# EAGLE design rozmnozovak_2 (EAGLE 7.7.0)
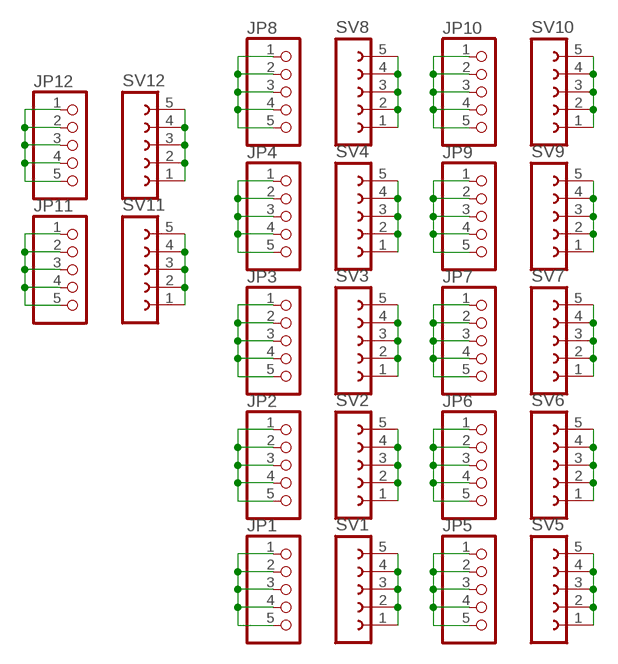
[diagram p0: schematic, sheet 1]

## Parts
JP1  PINHD-1X5  [1X05]
JP2  PINHD-1X5  [1X05]
JP3  PINHD-1X5  [1X05]
JP4  PINHD-1X5  [1X05]
JP5  PINHD-1X5  [1X05]
JP6  PINHD-1X5  [1X05]
JP7  PINHD-1X5  [1X05]
JP8  PINHD-1X5  [1X05]
JP9  PINHD-1X5  [1X05]
JP10  PINHD-1X5  [1X05]
JP11  PINHD-1X5  [1X05]
JP12  PINHD-1X5  [1X05]
SV1  FE05-1  [FE05-1]
SV2  FE05-1  [FE05-1]
SV3  FE05-1  [FE05-1]
SV4  FE05-1  [FE05-1]
SV5  FE05-1  [FE05-1]
SV6  FE05-1  [FE05-1]
SV7  FE05-1  [FE05-1]
SV8  FE05-1  [FE05-1]
SV9  FE05-1  [FE05-1]
SV10  FE05-1  [FE05-1]
SV11  FE05-1  [FE05-1]
SV12  FE05-1  [FE05-1]

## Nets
N$1: SV4.1 SV4.2 SV4.3 SV4.4 SV4.5
N$2: SV3.1 SV3.2 SV3.3 SV3.4 SV3.5
N$3: SV2.1 SV2.2 SV2.3 SV2.4 SV2.5
N$4: SV1.1 SV1.2 SV1.3 SV1.4 SV1.5
N$5: JP4.1 JP4.2 JP4.3 JP4.4 JP4.5
N$6: JP3.1 JP3.2 JP3.3 JP3.4 JP3.5
N$7: JP2.1 JP2.2 JP2.3 JP2.4 JP2.5
N$8: JP1.1 JP1.2 JP1.3 JP1.4 JP1.5
N$9: SV9.1 SV9.2 SV9.3 SV9.4 SV9.5
N$10: SV7.1 SV7.2 SV7.3 SV7.4 SV7.5
N$11: SV6.1 SV6.2 SV6.3 SV6.4 SV6.5
N$12: SV5.1 SV5.2 SV5.3 SV5.4 SV5.5
N$13: JP9.1 JP9.2 JP9.3 JP9.4 JP9.5
N$14: SV8.1 SV8.2 SV8.3 SV8.4 SV8.5
N$15: JP8.1 JP8.2 JP8.3 JP8.4 JP8.5
N$16: JP7.1 JP7.2 JP7.3 JP7.4 JP7.5
N$17: JP6.1 JP6.2 JP6.3 JP6.4 JP6.5
N$18: JP5.1 JP5.2 JP5.3 JP5.4 JP5.5
N$19: SV10.1 SV10.2 SV10.3 SV10.4 SV10.5
N$20: JP10.1 JP10.2 JP10.3 JP10.4 JP10.5
N$21: SV11.1 SV11.2 SV11.3 SV11.4 SV11.5
N$22: JP11.1 JP11.2 JP11.3 JP11.4 JP11.5
N$23: SV12.1 SV12.2 SV12.3 SV12.4 SV12.5
N$24: JP12.1 JP12.2 JP12.3 JP12.4 JP12.5

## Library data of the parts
JP1-JP12 = pinhead:PINHD-1X5: PIN HEADER
SV1-SV12 = con-lsta:FE05-1: FEMALE HEADER; OC_FARNELL: unknown; OC_NEWARK: unknown

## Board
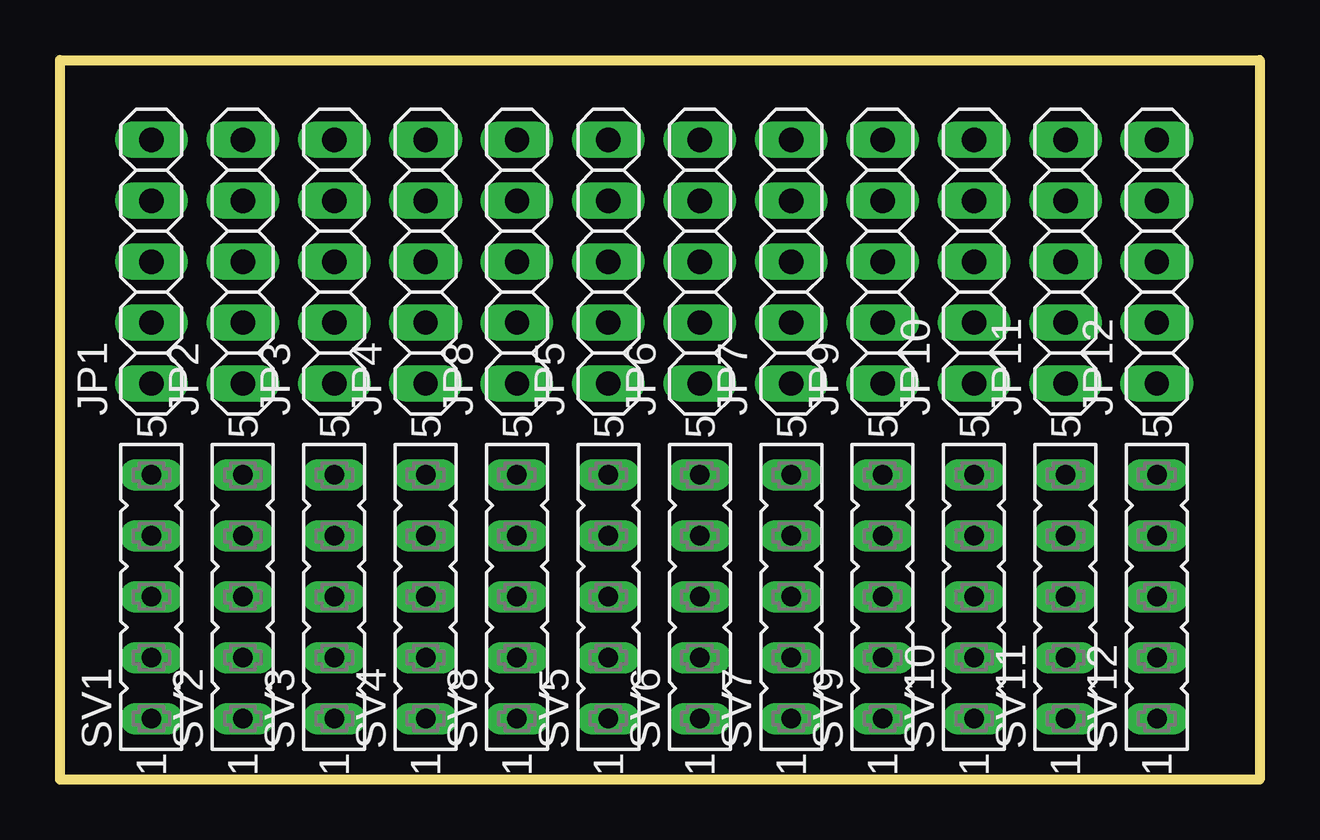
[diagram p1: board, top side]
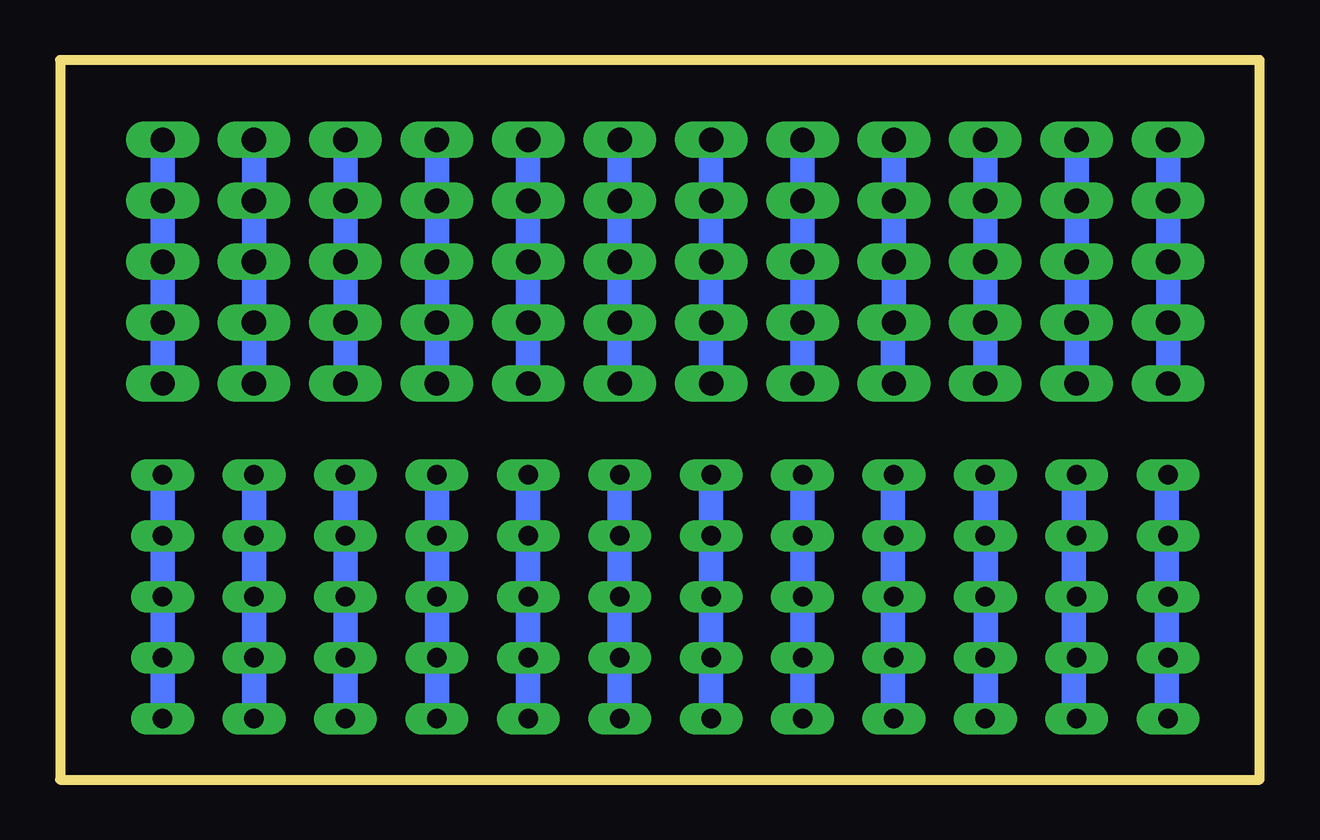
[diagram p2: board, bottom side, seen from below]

Size 50 x 30 mm. Coordinates in mm from the lower left corner, seen from the top.
Outline: 0,0 0,30 50,30 50,0 0,0
Copper layers (1*16): Top 0.035mm / dielectric 1.5mm / Bottom 0.035mm
Design rules "default": minimum track width 10mil, minimum drill 24mil, track to track 8mil, track to pad 8mil, pad to pad 8mil, via to via 8mil, smd to smd 8mil, copper to edge 40mil, drill to drill 8mil, minimum pad ring 10mil, minimum via ring 8mil, stop-mask expansion 4mil, vias tented up to drill 0mil, thermal gap 10mil

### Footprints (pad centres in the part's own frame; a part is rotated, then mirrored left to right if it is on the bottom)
1X05 = drill 1.016 long: 1 -5.08,0; 2 -2.54,0; 3 0,0; 4 2.54,0; 5 5.08,0
FE05-1 = drill 0.813 long: 1 -5.08,0; 2 -2.54,0; 3 0,0; 4 2.54,0; 5 5.08,0

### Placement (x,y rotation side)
JP1  3.81,21.59 90 top
JP2  7.62,21.59 90 top
JP3  11.43,21.59 90 top
JP4  15.24,21.59 90 top
JP5  22.86,21.59 90 top
JP6  26.67,21.59 90 top
JP7  30.48,21.59 90 top
JP8  19.05,21.59 90 top
JP9  34.29,21.59 90 top
JP10  38.1,21.59 90 top
JP11  41.91,21.59 90 top
JP12  45.72,21.59 90 top
SV1  3.81,7.62 90 top
SV2  7.62,7.62 90 top
SV3  11.43,7.62 90 top
SV4  15.24,7.62 90 top
SV5  22.86,7.62 90 top
SV6  26.67,7.62 90 top
SV7  30.48,7.62 90 top
SV8  19.05,7.62 90 top
SV9  34.29,7.62 90 top
SV10  38.1,7.62 90 top
SV11  41.91,7.62 90 top
SV12  45.72,7.62 90 top

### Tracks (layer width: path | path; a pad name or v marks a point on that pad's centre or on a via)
N$1
  Bottom 0.254: 15.29,2.74 SV4.1 | 15.29,5.03 SV4.2 15.29,5.26 | 15.29,7.77 SV4.3 15.29,7.54 | 15.29,10.06 SV4.4 15.29,10.29 | 15.29,12.57 SV4.5
  Bottom 1.016: 15.29,5.03 15.29,2.74 | 15.29,10.06 15.29,7.77 | 15.29,10.29 15.29,12.57 | 15.29,7.54 15.29,5.26
N$2
  Bottom 0.254: 11.4,2.74 SV3.1 | 11.4,5.03 SV3.2 11.4,5.26 | 11.4,7.77 SV3.3 11.4,7.54 | 11.4,10.06 SV3.4 11.4,10.29 | 11.4,12.57 SV3.5
  Bottom 1.016: 11.4,5.03 11.4,2.74 | 11.4,10.06 11.4,7.77 | 11.4,10.29 11.4,12.57 | 11.4,7.54 11.4,5.26
N$3
  Bottom 0.254: 7.75,2.74 SV2.1 | 7.75,5.03 SV2.2 7.75,5.26 | 7.75,7.77 SV2.3 7.75,7.54 | 7.75,10.06 SV2.4 7.75,10.29 | 7.75,12.57 SV2.5
  Bottom 1.016: 7.75,5.03 7.75,2.74 | 7.75,10.06 7.75,7.77 | 7.75,10.29 7.75,12.57 | 7.75,7.54 7.75,5.26
N$4
  Bottom 0.254: 3.86,2.74 SV1.1 | 3.86,5.03 SV1.2 3.86,5.26 | 3.86,7.77 SV1.3 3.86,7.54 | 3.86,10.06 SV1.4 3.86,10.29 | 3.86,12.57 SV1.5
  Bottom 1.016: 3.86,5.03 3.86,2.74 | 3.86,10.06 3.86,7.77 | 3.86,10.29 3.86,12.57 | 3.86,7.54 3.86,5.26
N$5
  Bottom 0.254: 15.29,16.69 JP4.1 | 15.29,18.75 JP4.2
  Bottom 1.016: JP4.5 JP4.4 JP4.3 JP4.2 | 15.29,18.75 15.29,16.69
N$6
  Bottom 1.016: JP3.5 JP3.4 JP3.3 JP3.2 JP3.1
N$7
  Bottom 1.016: JP2.5 JP2.4 JP2.3 JP2.2 JP2.1
N$8
  Bottom 1.016: JP1.5 JP1.4 JP1.3 JP1.2 JP1.1
N$9
  Bottom 1.016: SV9.5 SV9.4 SV9.3 SV9.2 SV9.1
N$10
  Bottom 1.016: SV7.5 SV7.4 SV7.3 SV7.2 SV7.1
N$11
  Bottom 1.016: SV6.5 SV6.4 SV6.3 SV6.2 SV6.1
N$12
  Bottom 1.016: SV5.5 SV5.4 SV5.3 SV5.2 SV5.1
N$13
  Bottom 1.016: JP9.5 JP9.4 JP9.3 JP9.2 JP9.1
N$14
  Bottom 1.016: SV8.5 SV8.4 SV8.3 SV8.2 SV8.1
N$15
  Bottom 1.016: JP8.5 JP8.4 JP8.3 JP8.2 JP8.1
N$16
  Bottom 1.016: JP7.1 JP7.2 JP7.3 JP7.4 JP7.5
N$17
  Bottom 1.016: JP6.5 JP6.4 JP6.3 JP6.2 JP6.1
N$18
  Bottom 1.016: JP5.5 JP5.4 JP5.3 JP5.2 JP5.1
N$19
  Bottom 1.016: SV10.5 SV10.4 SV10.3 SV10.2 SV10.1
N$20
  Bottom 1.016: JP10.5 JP10.4 JP10.3 JP10.2 JP10.1
N$21
  Bottom 1.016: SV11.5 SV11.4 SV11.3 SV11.2 SV11.1
N$22
  Bottom 1.016: JP11.5 JP11.4 JP11.3 JP11.2 JP11.1
N$23
  Bottom 1.016: SV12.5 SV12.4 SV12.3 SV12.2 SV12.1
N$24
  Bottom 1.016: JP12.5 JP12.4 JP12.3 JP12.2 JP12.1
